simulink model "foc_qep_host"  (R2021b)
settings: Solver=FixedStepDiscrete  StartTime=0.0  StopTime=Inf  RelTol=1e-3
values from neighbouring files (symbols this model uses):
  pmsm = mcb_SetPMSMMotorParameters('BLY171D')    [foc_qep_data.m]
undefined symbols (not defined in the file or in its folder): Serial
libraries: mcbhostblockslib x3

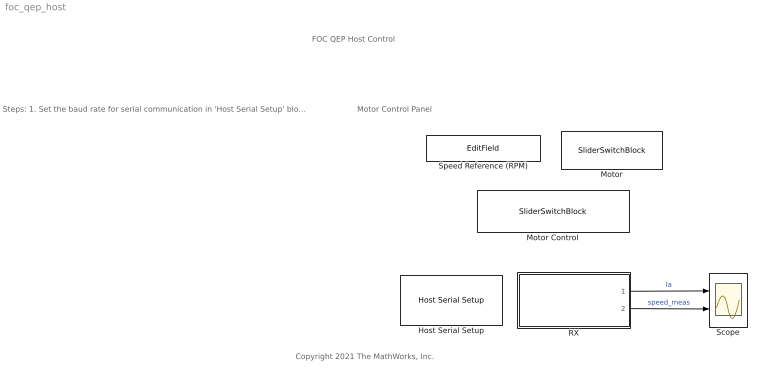
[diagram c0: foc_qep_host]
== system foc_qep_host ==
  note: FOC QEP Host Control
  note: Motor Control Panel
  note: Steps: 1. Set the baud rate for serial communication in 'Host Serial Setup' block. 2. Select the serial port in ' Serial 1 ' tab of ' Host Serial Setup ' block. 3. Use ' Motor Start / Stop ' switch to control the start and stop of the motor. 4. Use the ' Motor Control Open Loop / Closed Loop ' switch to switch between open loop and closed loop control. 4. Enter speed request in RPM using 'Speed Reference' edit box. Limit the reference speed to half of the rated speed while starting the motor in open loop. 5. Observe the Ia and measured speed signals on the scope.
  note: Copyright 2021 The MathWorks, Inc.
  Host Serial Setup : mcbhostblockslib/Host Serial Setup  Priority=-99  comPortSer1='Please_select_a_port'  baudRateA=4000000  charLenA=8  stopBitA=1  parityA=none  timeoutA=2.0  ByteOrderA=LittleEndian  comPortSer2='Please_select_a_port'  baudRateB=115200  charLenB=8  stopBitB=1  parityB=none  timeoutB=1.0  ByteOrderB=LittleEndian  comPortSer3='Please_select_a_port'  baudRateC=115200  charLenC=8  stopBitC=1  parityC=none  timeoutC=1.0  ByteOrderC=LittleEndian  comPortSer4='Please_select_a_port'  baudRateD=115200  charLenD=8  stopBitD=1  parityD=none  timeoutD=1.0  ByteOrderD=LittleEndian
  Motor : SliderSwitchBlock  LabelPosition=Hide
  Motor Control : SliderSwitchBlock  LabelPosition=Hide
  RX : Subsystem
  Scope : Scope  NumInputPorts=2
  Speed Reference (RPM) : EditField  LabelPosition=Hide  ShowInitialText=on  Alignment=Center
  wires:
  RX/1(Ia_pu) -> Scope/1  "Ia"
  RX/2(speed_meas_pu) -> Scope/2  "speed_meas"

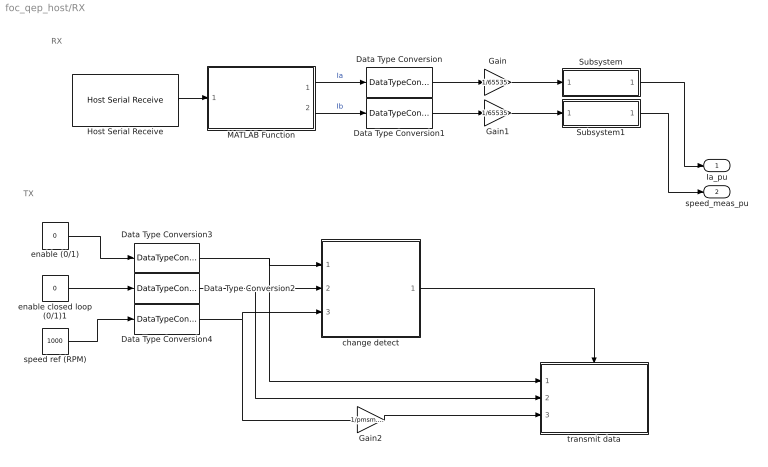
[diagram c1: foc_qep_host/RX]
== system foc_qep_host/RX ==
  note: TX
  note: RX
  Data Type Conversion{,1..4} (5 alike) : DataTypeConversion  OutDataTypeStr=single
  Gain : Gain  Gain=1/65535  OutDataTypeStr=single
  Gain1 : Gain  Gain=1/65535  OutDataTypeStr=single
  Gain2 : Gain  Gain=1/pmsm.N_base  OutDataTypeStr=single
  Host Serial Receive : mcbhostblockslib/Host Serial Receive  serialCon=Serial 1  dataHead='ss'  dataTail='ee'  dataType=uint16  dataDim=[200 2]  initValue=2000  errOption=Output custom value  errValue=4000  sampleTime=200 * 50e-6  outputStatus=off  blockingMode=on
  MATLAB Function : MATLAB Function  TreatAsAtomicUnit=on
  Subsystem : Subsystem
  Subsystem1 : Subsystem
  change detect : Subsystem
  enable (0/1) : Constant  Value=0  OutDataTypeStr=boolean  SampleTime=-1
  enable closed loop (0/1)1 : Constant  Value=0  OutDataTypeStr=boolean  SampleTime=-1
  speed ref (RPM) : Constant  Value=1000  OutDataTypeStr=single  SampleTime=-1
  transmit data : Subsystem  TreatAsAtomicUnit=on
  Ia_pu : Outport
  speed_meas_pu : Outport  Port=2
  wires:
  Subsystem/1(Out1) -> Ia_pu/1
  Subsystem1/1(Out1) -> speed_meas_pu/1
  Data Type Conversion/1 -> Gain/1
  Data Type Conversion1/1 -> Gain1/1
  Gain/1 -> Subsystem/1(In1)
  MATLAB Function/1(Output1) -> Data Type Conversion/1  "Ia"
  Gain1/1 -> Subsystem1/1(In1)
  Host Serial Receive/1 -> MATLAB Function/1(Input)
  MATLAB Function/2(Output2) -> Data Type Conversion1/1  "Ib"
  Gain2/1 -> transmit data/3(speed_ref_rpm)
  enable (0/1)/1 -> Data Type Conversion3/1
  Data Type Conversion2/1 -> transmit data/2(enable_cl), change detect/2(enable_cl)
  enable closed loop (0/1)1/1 -> Data Type Conversion2/1
  Data Type Conversion4/1 -> Gain2/1, change detect/3(speed_ref_rpm)
  Data Type Conversion3/1 -> transmit data/1(enable), change detect/1(enable)
  change detect/1(isChange) -> transmit data/Enable
  speed ref (RPM)/1 -> Data Type Conversion4/1

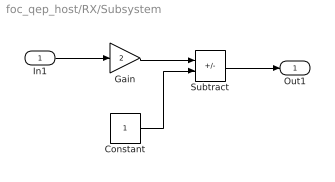
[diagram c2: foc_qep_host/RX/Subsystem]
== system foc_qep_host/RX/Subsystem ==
  In1 : Inport
  Constant : Constant
  Gain : Gain  Gain=2
  Subtract : Sum  Inputs=+-
  Out1 : Outport
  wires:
  In1/1 -> Gain/1
  Gain/1 -> Subtract/1
  Subtract/1 -> Out1/1
  Constant/1 -> Subtract/2

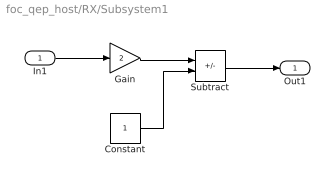
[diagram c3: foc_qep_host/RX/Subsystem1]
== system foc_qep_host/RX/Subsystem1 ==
  In1 : Inport
  Constant : Constant
  Gain : Gain  Gain=2
  Subtract : Sum  Inputs=+-
  Out1 : Outport
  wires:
  In1/1 -> Gain/1
  Gain/1 -> Subtract/1
  Subtract/1 -> Out1/1
  Constant/1 -> Subtract/2

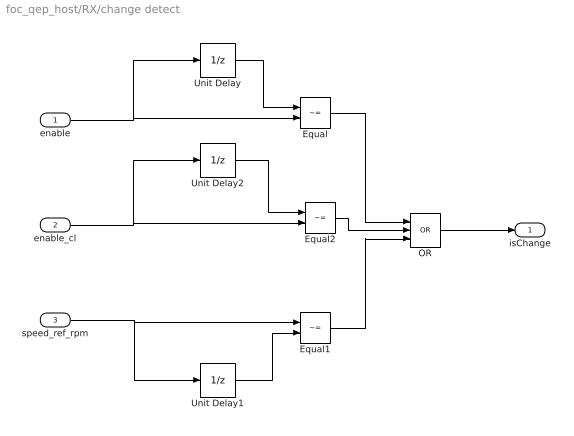
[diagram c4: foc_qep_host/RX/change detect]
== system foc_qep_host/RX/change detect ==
  enable : Inport
  enable_cl : Inport  Port=2
  speed_ref_rpm : Inport  Port=3
  Equal : RelationalOperator  Operator=~=  OutDataTypeStr=boolean  RndMeth=Simplest
  Equal1 : RelationalOperator  Operator=~=  OutDataTypeStr=boolean  RndMeth=Simplest
  Equal2 : RelationalOperator  Operator=~=  OutDataTypeStr=boolean  RndMeth=Simplest
  OR : Logic  Operator=OR  Inputs=3  AllPortsSameDT=off  OutDataTypeStr=boolean
  Unit Delay : UnitDelay  SampleTime=-1  HasFrameUpgradeWarning=on
  Unit Delay1 : UnitDelay  SampleTime=-1  HasFrameUpgradeWarning=on
  Unit Delay2 : UnitDelay  SampleTime=-1  HasFrameUpgradeWarning=on
  isChange : Outport
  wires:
  Unit Delay/1 -> Equal/1
  enable/1 -> Equal/2, Unit Delay/1
  speed_ref_rpm/1 -> Unit Delay1/1, Equal1/1
  Unit Delay1/1 -> Equal1/2
  OR/1 -> isChange/1
  Equal/1 -> OR/1
  Equal1/1 -> OR/3
  Equal2/1 -> OR/2
  enable_cl/1 -> Unit Delay2/1, Equal2/2
  Unit Delay2/1 -> Equal2/1

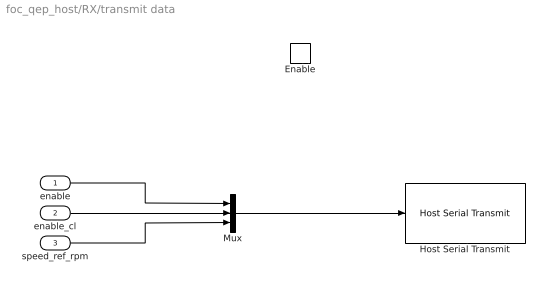
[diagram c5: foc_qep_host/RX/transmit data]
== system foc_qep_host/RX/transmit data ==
  enable : Inport
  enable_cl : Inport  Port=2
  speed_ref_rpm : Inport  Port=3
  Enable : EnablePort
  Host Serial Transmit : mcbhostblockslib/Host Serial Transmit  serialCon=Serial 1  header=''  tail=''  enableBlockingMode=off
  Mux : Mux  Inputs=3
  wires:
  enable/1 -> Mux/1
  Mux/1 -> Host Serial Transmit/1
  speed_ref_rpm/1 -> Mux/3
  enable_cl/1 -> Mux/2

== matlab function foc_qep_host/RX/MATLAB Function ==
function [ Output1, Output2] = unBuf(Input)

Output1 = Input(:, 1);
Output2 = Input(:, 2);
end
